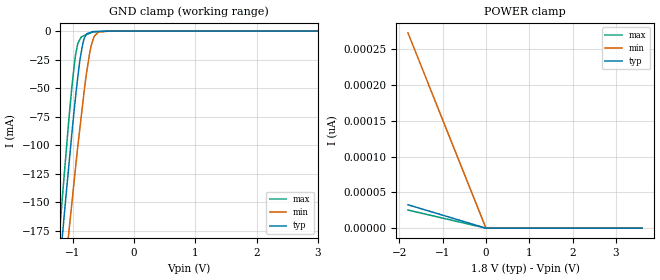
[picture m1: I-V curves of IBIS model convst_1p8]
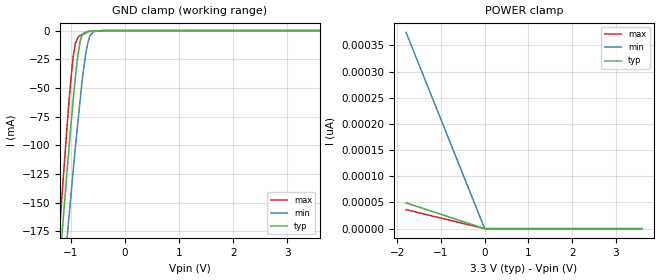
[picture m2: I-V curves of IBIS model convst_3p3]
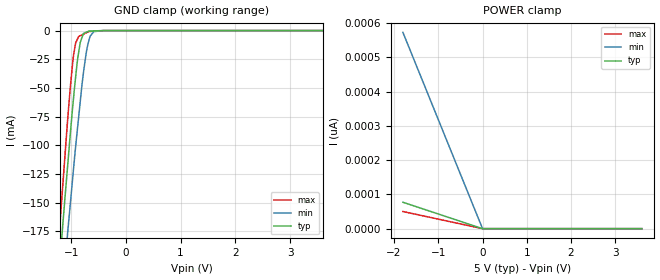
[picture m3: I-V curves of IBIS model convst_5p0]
|Texas Instruments Incorporated
| 16-Channel, 16-Bit, 1-MSPS, Dual, Simultaneous Sampling ADC With
| Integrated Analog Front End
| Marketing Part # : ADS8686S
| Digital Voltage Range : 1.71V-5.25V
| Package-type: LQFP
| #pins/pkg drawing : 80-pin PZA
[IBIS Ver] 4.1
[File name] ads8686s.ibs
[File Rev] 1.0
[Date] 12/13/2019
[Source]
| Texas Instruments Incorporated.
| 12500 TI Blvd
| Dallas, TX -75243
[Notes] Revision History:
| Rev 1.0: 02/18/2019
| - Initial version of the model
| - Model generated from simulations in TISPICE/SPECTRE
| - C_comp although listed in numerical order of value are
| obtained from varying PVT conditions. For PVT conditions for
| each specific value refer the buffer description under
| respective [Model]. IBIS model user is responsible for using
| appropriate C_comp to simulate for Signal Integrity.
| - Warnings regarding combined Non-monotonicity of various models have been
| reviewed and considered minor and can be ignored.
| - Model names with a trailing _1p8 contain the model for
| 1.8V operation. Model names with a trailing _3p3 contain the model
| for 3.3V operation.Model names with a trailing _5p0 contain the model
| for 5.0V operation
[Disclaimer]
| This model is designed as an aid for customers of Texas Instruments.
| TI and its licensors and suppliers make no warranties, either expressed
| or implied, with respect to this model, including the warranties of
| merchantability or fitness for a particular purpose. The model is
| provided solely on an "as is" basis. The entire risk as to its quality
| and performance is with the customer.
| This model is subject to change without notice. Texas Instruments
| Incorporated is not responsible for updating this model.
[Copyright]
(C) Copyright 2019 Texas Instruments Incorporated. All rights reserved.
|ADS8686S
[Component] ADS8686S
[Manufacturer] Texas Instruments Incorporated
[Package] |LQFP (PZA) 80-pin
| variable typ min max
R_pkg 0.088 0.043 0.112
L_pkg 4.14nH 2.78nH 5.13nH
C_pkg 0.006pF 0.0048pF 0.0072pF
|pin number (pin name) mapping to model name
[Pin]  signal_name   model_name   R_pin   L_pin   C_pin
1   AIN_4BGND   nc   NA   NA   NA
2   AIN_4B   nc   NA   NA   NA
3   AIN_5BGND   nc   NA   NA   NA
4   AIN_5B   nc   NA   NA   NA
5   AGND   gnd   NA   NA   NA
6   AVDD   power   NA   NA   NA
7   AIN_6B   nc   NA   NA   NA
8   AIN_6BGND   nc   NA   NA   NA
9   AIN_7B   nc   NA   NA   NA
10   AIN_7BGND   nc   NA   NA   NA
11   AIN_7AGND   nc   NA   NA   NA
12   AIN_7A   nc   NA   NA   NA
13   AIN_6AGND   nc   NA   NA   NA
14   AIN_6A   nc   NA   NA   NA
15   AVDD   power   NA   NA   NA
16   AGND   gnd   NA   NA   NA
17   AIN_5A   nc   NA   NA   NA
18   AIN_5AGND   nc   NA   NA   NA
19   AIN_4A   nc   NA   NA   NA
20   AIN_4AGND   nc   NA   NA   NA
21   AIN_3AGND   nc   NA   NA   NA
22   AIN_3A   nc   NA   NA   NA
23   AIN_2AGND   nc   NA   NA   NA
24   AIN_2A   nc   NA   NA   NA
25   AIN_1AGND   nc   NA   NA   NA
26   AIN_1A   nc   NA   NA   NA
27   AIN_0AGND   nc   NA   NA   NA
28   AIN_0A   nc   NA   NA   NA
29   AGND   gnd   NA   NA   NA
30   AVDD   power   NA   NA   NA
31   REFCAP   nc   NA   NA   NA
32   REFGND   gnd   NA   NA   NA
33   REFIO   nc   NA   NA   NA
34   REFIO_GND   gnd   NA   NA   NA
35   REFSEL   convst   NA   NA   NA
36   RESETZ   convst   NA   NA   NA
37   SEQEN   convst   NA   NA   NA
38   HW_RNGSEL1   convst   NA   NA   NA
39   HW_RNGSEL0   convst   NA   NA   NA
40   SER_PARZ   convst   NA   NA   NA
41   DB0   db15   NA   NA   NA
42   DB1   db15   NA   NA   NA
43   DB2   db15   NA   NA   NA
44   DB3   db15   NA   NA   NA
45   DB4_SER1WZ   db15   NA   NA   NA
46   DB5_CRCEN   db15   NA   NA   NA
47   DB6   db15   NA   NA   NA
48   DB7   db15   NA   NA   NA
49   DVDD   power   NA   NA   NA
50   DGND   gnd   NA   NA   NA
51   REGGNDD   gnd   NA   NA   NA
52   REGCAPD   power   NA   NA   NA
53   DB8_FLTEN   db15   NA   NA   NA
54   DB9_BYTESEL   db15   NA   NA   NA
55   DB10_SDI   db15   NA   NA   NA
56   DB11_SDOB   db15   NA   NA   NA
57   DB12_SDOA   db15   NA   NA   NA
58   DB13_OS0   db15   NA   NA   NA
59   DB14_OS1   db15   NA   NA   NA
60   DB15_OS2   db15   NA   NA   NA
61   WRZ_BURST   convst   NA   NA   NA
62   SCLK_RDZ   convst   NA   NA   NA
63   CSZ   convst   NA   NA   NA
64   CHSEL0   convst   NA   NA   NA
65   CHSEL1   convst   NA   NA   NA
66   CHSEL2   convst   NA   NA   NA
67   BUSY   busy   NA   NA   NA
68   CONVST   convst   NA   NA   NA
69   REGGND   gnd   NA   NA   NA
70   REGCAP   power   NA   NA   NA
71   AVDD   power   NA   NA   NA
72   AGND   gnd   NA   NA   NA
73   AIN_0B   nc   NA   NA   NA
74   AIN_0BGND   nc   NA   NA   NA
75   AIN_1B   nc   NA   NA   NA
76   AIN_1BGND   nc   NA   NA   NA
77   AIN_2B   nc   NA   NA   NA
78   AIN_2BGND   nc   NA   NA   NA
79   AIN_3B   nc   NA   NA   NA
80   AIN_3BGND   nc   NA   NA   NA
|   Model Selectors
[Model Selector] convst
convst_1p8   1.8V  digital Input
convst_3p3   3.3V  digital Input
convst_5p0   5.0V  digital Input
[Model Selector] busy
busy_1p8   1.8V  digital Output
busy_3p3   3.3V  digital Output
busy_5p0   5.0V  digital Output
[Model Selector] db15
db15_1p8   1.8V  digital I/O
db15_3p3   3.3V  digital I/O
db15_5p0   5.0V  digital I/O
| Models and submodels in the file (9): convst_1p8 (Input), convst_3p3 (Input), convst_5p0 (Input), busy_1p8 (3-state), busy_3p3 (3-state), busy_5p0 (3-state), db15_1p8 (I/O), db15_3p3 (I/O), db15_5p0 (I/O)
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|   convst_1p8 Model
[Model]   convst_1p8
Model_type   Input
Vinl = 0.54
Vinh = 1.26
|   typ   min   max
C_comp   0.870pF   0.866pF   0.882pF
[Voltage Range]   1.8   1.71   1.89
[Temperature Range]   27   125   -40
[Power Clamp Reference]   1.8   1.71   1.89
[GND Clamp Reference]   0   0   0
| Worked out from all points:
|   GND clamp passes 1 mA (typ) near -0.70 V on its own axis
[GND Clamp]
|   Voltage   I(typ)   I(min)   I(max)
-1.8V     -575.1mA   -590.1mA   -589.5mA
-1.221V   -211.2mA   -262.2mA   -180.8mA
-1.167V   -178.5mA   -232.5mA   -144.6mA
-1.059V   -115.6mA   -174.2mA   -75.37mA
-952.5mV  -57.21mA   -118.9mA   -20.52mA
-917.8mV  -40.79mA   -101.3mA   -10.96mA
-853.4mV  -16.41mA   -71.37mA   -4.885mA
-809.9mV  -6.098mA   -51.12mA   -3.9mA
-714mV    -1.236mA   -16.77mA   -1.732mA
-657.5mV  -428.2uA   -5.673mA   -745.9uA
-583.1mV  -291.6uA   -884.3uA   -530.6uA
3.6V      0A         0A         0A
[POWER Clamp]
|   Voltage   I(typ)   I(min)   I(max)
-1.8V     32.7pA     272.9pA    25.34pA
0V        0A         0A         0A
3.6V      0A         0A         0A
|   convst_3p3 Model
[Model]   convst_3p3
Model_type   Input
Vinl = 0.99
Vinh = 2.31
|   typ   min   max
C_comp   0.786pF   0.783pF   0.797pF
[Voltage Range]   3.3   3.135   3.465
[Temperature Range]   27   125   -40
[Power Clamp Reference]   3.3   3.135   3.465
[GND Clamp Reference]   0   0   0
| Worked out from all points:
|   GND clamp passes 1 mA (typ) near -0.70 V on its own axis
[GND Clamp]
|   Voltage   I(typ)   I(min)   I(max)
-1.8V     -575.1mA   -590.1mA   -589.5mA
-1.221V   -211.2mA   -262.2mA   -180.8mA
-1.167V   -178.5mA   -232.5mA   -144.6mA
-1.059V   -115.6mA   -174.2mA   -75.37mA
-952.5mV  -57.21mA   -118.9mA   -20.52mA
-917.8mV  -40.79mA   -101.3mA   -10.96mA
-853.4mV  -16.41mA   -71.37mA   -4.885mA
-809.9mV  -6.098mA   -51.12mA   -3.9mA
-714mV    -1.236mA   -16.77mA   -1.732mA
-657.5mV  -428.2uA   -5.673mA   -745.9uA
-583.1mV  -291.6uA   -884.3uA   -530.6uA
3.6V      0A         0A         0A
[POWER Clamp]
|   Voltage   I(typ)   I(min)   I(max)
-1.8V     49.23pA    374.9pA    36.27pA
0V        0A         0A         0A
3.6V      0A         0A         0A
|   convst_5p0 Model
[Model]   convst_5p0
Model_type   Input
Vinl = 1.5
Vinh = 3.5
|   typ   min   max
C_comp   0.727pF   0.724pF   0.737pF
[Voltage Range]   5   4.75   5.25
[Temperature Range]   27   125   -40
[Power Clamp Reference]   5   4.75   5.25
[GND Clamp Reference]   0   0   0
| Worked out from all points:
|   GND clamp passes 1 mA (typ) near -0.70 V on its own axis
[GND Clamp]
|   Voltage   I(typ)   I(min)   I(max)
-1.8V     -575.1mA   -590.1mA   -589.5mA
-1.221V   -211.2mA   -262.2mA   -180.8mA
-1.167V   -178.5mA   -232.5mA   -144.6mA
-1.059V   -115.6mA   -174.2mA   -75.37mA
-952.5mV  -57.21mA   -118.9mA   -20.52mA
-917.8mV  -40.79mA   -101.3mA   -10.96mA
-853.4mV  -16.41mA   -71.37mA   -4.885mA
-777mV    -2.831mA   -37.62mA   -3.157mA
-714mV    -1.236mA   -16.77mA   -1.732mA
-657.5mV  -428.2uA   -5.673mA   -745.9uA
-583.1mV  -291.6uA   -884.3uA   -530.6uA
3.6V      0A         0A         0A
[POWER Clamp]
|   Voltage   I(typ)   I(min)   I(max)
-1.8V     77.1pA     572.9pA    50.02pA
0V        0A         0A         0A
3.6V      0A         0A         0A
